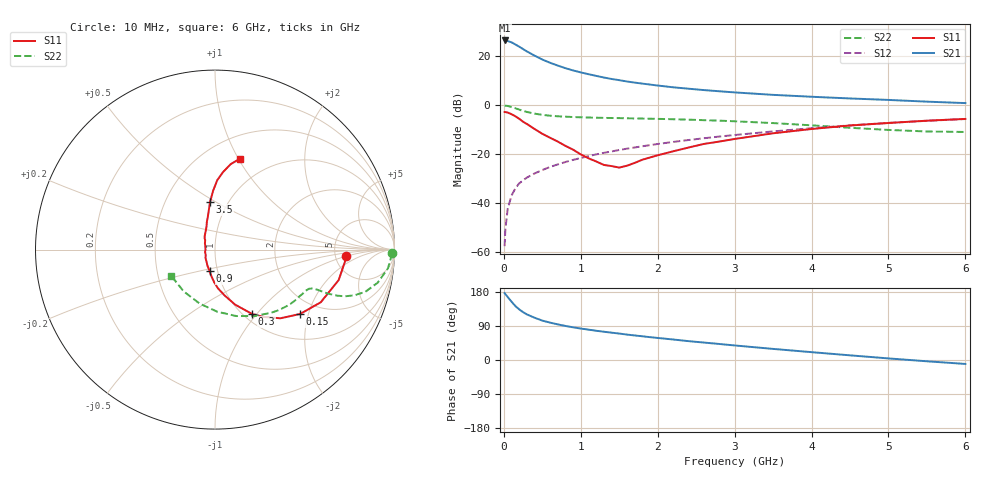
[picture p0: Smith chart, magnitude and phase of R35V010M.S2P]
! SIEMENS Small Signal Semiconductors
! BFR181
! Si NPN RF Bipolar Junction Transistor in SOT23
! VCE = 5 V  IC = 10 mA
! Common Emitter S-Parameters:  May  1996
# GHz  S  MA  R  50
!  f  S11  S21  S12  S22
! GHz  MAG  ANG  MAG  ANG  MAG  ANG  MAG  ANG
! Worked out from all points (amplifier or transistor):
!   36 points, 10 MHz to 6 GHz, reference 50 ohm
!   highest |S21| = 26.6 dB at 10 MHz (marker M1)
!   |S21| within 3 dB of that: start of sweep to 223 MHz
!   unconditionally stable (mu >= 1): 819.1 MHz to 2.697 GHz
!   at 250 MHz: K = 0.60, MSG = 26.9 dB, |S12| = -30.8 dB
!   at 1.4 GHz: K = 1.05, MAG = 13.4 dB, |S12| = -18.9 dB
!   at 6 GHz: K = 0.86, MSG = 3.3 dB, |S12| = -5.6 dB
!   S11 on the Smith chart (normalised r, x): 10 MHz: 6.22, -0.98; 150 MHz: 1.60, -1.77; 300 MHz: 1.09, -0.95; 900 MHz: 0.92, -0.22; 3.5 GHz: 0.82, +0.47; 6 GHz: 0.72, +1.02
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0.01  0.729 -2.9  21.31 176.6  0.0013 86.7  0.985 -1.2
0.02  0.727 -5.3  21.03 173.9  0.0029 88.0  0.9821 -2.5
0.05  0.7098 -13.8  20.75 166.2  0.0075 84.8  0.9694 -6.2
0.1  0.6582 -26.5  19.5 153.9  0.0142 79.6  0.925 -11.5
0.15  0.5945 -37.1  17.63 142.3  0.0199 72.7  0.8696 -15.7
0.2  0.5285 -46.4  15.89 133.6  0.0252 70.9  0.8165 -18.2
0.25  0.4608 -54.4  14.2 126.2  0.029 69.4  0.7684 -19.8
0.3  0.4143 -60.0  12.69 120.3  0.0331 69.1  0.7301 -20.6
0.4  0.3266 -69.9  10.4 111.5  0.0402 68.4  0.6754 -21.3
0.5  0.2607 -78.2  8.657 104.0  0.0472 68.8  0.6373 -21.4
0.6  0.2166 -85.6  7.449 98.7  0.0545 69.3  0.6127 -21.4
0.7  0.1811 -91.6  6.522 94.0  0.0615 69.6  0.5953 -21.6
0.9  0.1235 -103.9  5.183 86.2  0.0762 70.0  0.5749 -22.2
1.1  0.0821 -125.1  4.34 80.1  0.0909 69.9  0.5616 -23.4
1.3  0.06 -149.4  3.71 74.6  0.1062 69.7  0.5522 -24.9
1.6  0.0578 159.0  3.075 67.1  0.1293 68.5  0.5421 -27.9
2.2  0.114 117.3  2.34 54.1  0.1775 65.2  0.5183 -35.6
2.8  0.1807 103.1  1.939 42.3  0.229 60.9  0.4847 -44.8
3.5  0.267 95.9  1.637 29.3  0.2919 54.6  0.432 -58.9
4.5  0.3861 88.2  1.381 12.3  0.388 43.9  0.3465 -87.8
5.5  0.484 79.6  1.188 -3.4  0.4813 31.2  0.291 -126.8
6  0.5262 74.6  1.11 -10.4  0.5235 24.3  0.2842 -148.7
